FUNCTION FC 1 : VOID
TITLE =
VERSION : 0.1


VAR_INPUT
  S0 : BOOL ;
  S1 : BOOL ;
  S2 : BOOL ;
  S3 : BOOL ;
  S4 : BOOL ;
  F3 : BOOL ;
END_VAR
VAR_OUTPUT
  K1 : BOOL ;
  K2 : BOOL ;
END_VAR
BEGIN
NETWORK
TITLE =
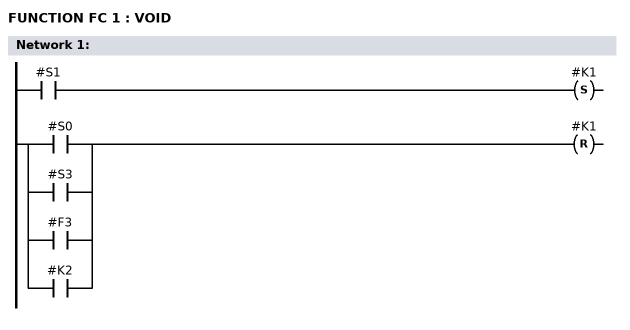
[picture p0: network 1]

      U     #S1;
      S     #K1;
      O     #S0;
      O     #S3;
      O     #F3;
      O     #K2;
      R     #K1;

END_FUNCTION

